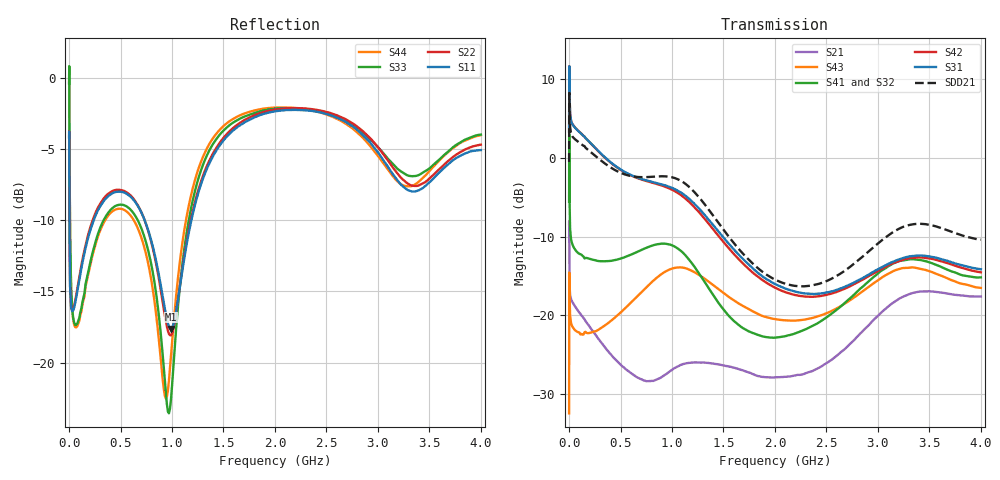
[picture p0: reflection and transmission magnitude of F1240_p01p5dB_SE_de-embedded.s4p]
! Integrated Device Technology
! Corporate Headquarters
! 6024 Silver Creek Valley Road
! San Jose, CA 95138  USA
! Phone:  1-408-284-8200
! Toll Free:  1-800-223-1366
! Webpage:  http://www.idt.com/
! Timing and RF Division
! 515 Groton Road, Suite 102
! Westford, MA 01886-6024
! Device:  F1240
! Description: Dual Intermediate Frequency Digital Variable Gain Amplifier
! Frequency:  10.0 -  500.00 MHz
! Package:  5x5 mm QFN Plastic Package: 32 pin
! Ports:  8 RF, 20 DC
!  Pin  1  = GA3 / Data  Pin 17  = RF OUT_B+
!  Pin  2  = GA4 / CLK  Pin 18  = RF OUT_B-
!  Pin  3  = GA5  Pin 19  = STBY_B
!  Pin  4  = VMODE  Pin 20  = Ground
!  Pin  5  = No Connect  Pin 21  = Ground
!  Pin  6  = GB5  Pin 22  = STB_A
!  Pin  7  = GB4  Pin 23  = RF OUT_A-  = Port 4
!  Pin  8  = GB3  Pin 24  = RF OUT_A+  = Port 3
!  Pin  9  = GB2  Pin 25  = GA0
!  Pin 10  = GB1  Pin 26  = ISET_A
!  Pin 11  = RF IN_B+  Pin 27  = VCC
!  Pin 12  = RF IN_B-  Pin 28  = Ground
!  Pin 13  = Ground  Pin 29  = RF IN_A-  = Port 2
!  Pin 14  = VCC  Pin 30  = RF IN_A+  = Port 1
!  Pin 15  = ISET_B  Pin 31  = GA1
!  Pin 16  = GB0  Pin 32  = GA2 / CSb
! Gain  = +19.5 dB
! State  = 1
! Voltage  = +5.00 V
! Current  = 85.292 mA (one channel only)
! Temperture  =  +25 C
! Test Date  =  2017-10-18
! Board  =  EB4031
! Data:  The device was measured on a custom evaluation board which has
!  individual transmission lines to the RF pins.  Data was collected
!  using a calibrated network analyzer.  The evaluation board was
!  de-embedded using Automatic Fixture Removal.
!  The reference plane is the edge of the package pin.
!  Only Channel A was measured.
!  This data is in single-ended operation.  If your needs are balanced
!  or differential S-parameters then this file needs to be used a
!  linear simulator.
! File Date:  2017-11-10  MJV
! Note:
!  Integrated Device Technology supplies this data as a sample of measured
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# Hz S dB R 100
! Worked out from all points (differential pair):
!   410 points, 500 kHz to 4 GHz, reference 100 ohm
!   strongest paths, dB at 500 kHz, 930 MHz, 1.96 GHz, 2.98 GHz, 4 GHz:
!     S31: 3.4, -3.5, -15.7, -14.3, -14.1
!     S42: 3.4, -3.6, -16.2, -14.5, -14.5
!     S41: -5.6, -10.9, -22.8, -14.9, -15.2
!     S32: -5.5, -11.1, -22.8, -15.3, -15.7
!     S43: -32.4, -14.5, -20.4, -15.7, -16.5
!     S21: -8.4, -27.5, -27.9, -20.3, -17.6
!   taken as a pair (ports 1,2 in; 3,4 out), SDD21 dB: -0.5, -2.3, -15.2, -11.1, -10.4
!   lowest |S11| = -17.6 dB at 990 MHz (marker M1), VSWR 1.30, Z = 78.3 - j8.86 ohm
!   |S11| at or under -10 dB: 4.048 MHz to 238.9 MHz (234.9 MHz wide, 193 % of centre); 734.9 MHz to 1.188 GHz (452.8 MHz wide, 47.1 % of centre)
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500000  -4.15 -5.6  -8.38 -5.7  -29.57 81.5  -38.35 79.1
        -8.39 -5.8  -4.15 -5.5  -38.38 78.2  -29.55 82.6
        3.37 -106.6  -5.53 -108.3  -0.35 1.0  -32.43 -50.7
        -5.55 -107.2  3.35 -105.5  -32.43 -50.8  -0.36 3.3
2500000  -6.60 -46.0  -12.06 -43.5  -19.09 26.1  -29.69 2.0
         -12.07 -43.5  -6.57 -46.0  -29.65 1.8  -19.09 26.4
         11.01 178.7  0.78 156.2  -0.93 -56.7  -14.62 -154.6
         0.74 156.4  11.00 179.0  -14.61 -154.6  -0.98 -56.4
4500000  -10.72 -51.1  -15.77 -34.3  -19.20 10.5  -32.23 -11.3
         -15.78 -34.3  -10.68 -51.5  -32.20 -11.5  -19.20 10.6
         8.30 162.3  -4.69 139.3  -5.11 -82.6  -17.15 174.7
         -4.74 139.4  8.30 162.4  -17.13 174.6  -5.17 -82.6
1.7e8  -11.64 -110.2  -20.88 -53.0  -21.31 -44.4  -35.66 -24.3
       -20.89 -52.9  -11.43 -111.6  -35.71 -23.9  -21.33 -44.6
       2.40 116.6  -12.72 77.4  -14.16 -139.0  -22.28 105.9
       -12.69 77.3  2.40 115.8  -22.22 105.4  -14.32 -138.7
5.2e8  -8.00 -164.1  -26.48 -107.3  -22.88 -108.8  -33.18 -72.9
       -26.48 -106.5  -7.89 -165.7  -33.33 -70.8  -23.06 -109.2
       -1.61 25.3  -12.79 -48.7  -8.90 -171.1  -19.59 9.4
       -12.70 -49.9  -1.66 24.0  -19.39 9.2  -9.21 -171.5
9.9e8  -17.64 -154.9  -27.27 -143.8  -21.92 150.5  -30.39 -164.2
       -26.99 -146.7  -18.09 -152.8  -30.42 -158.3  -22.49 149.2
       -3.74 -90.4  -11.23 166.7  -22.58 -126.7  -14.36 -113.0
       -11.04 163.0  -3.96 -92.9  -14.09 -113.3  -19.53 -111.9
4e9  -5.05 -140.9  -17.63 104.3  -24.06 -44.1  -25.01 -27.7
     -17.59 104.1  -4.67 -139.2  -25.89 -12.3  -25.81 -37.4
     -14.14 37.8  -15.66 -66.4  -3.95 -134.5  -17.88 66.9
     -15.16 -79.9  -14.52 43.7  -16.50 57.8  -4.00 -144.1
